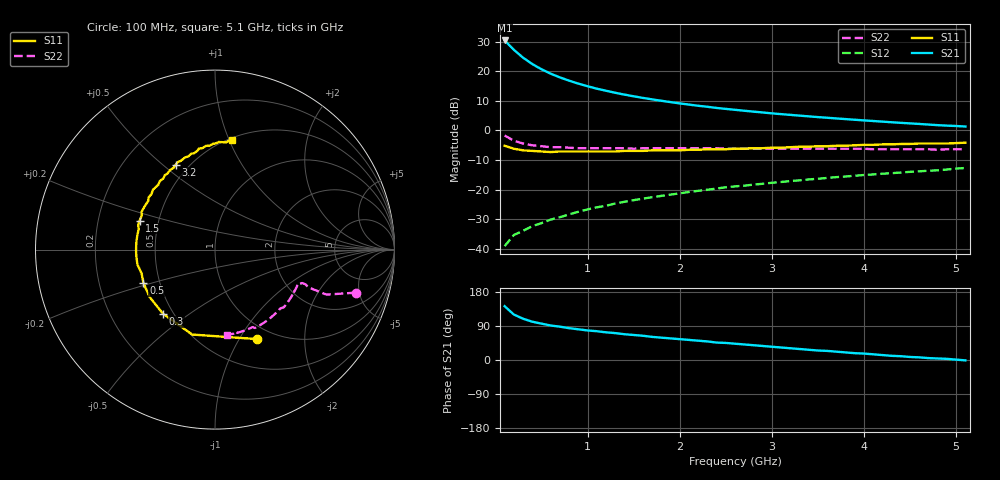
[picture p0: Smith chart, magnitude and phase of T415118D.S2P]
!AT-41511
!S-PARAMETERS at Vce=8V  Ic=25mA.  LAST UPDATED 01-25-95
# ghz s ma r 50
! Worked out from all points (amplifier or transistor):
!   51 points, 100 MHz to 5.1 GHz, reference 50 ohm
!   highest |S21| = 30.4 dB at 100 MHz (marker M1)
!   |S21| within 3 dB of that: start of sweep to 195.3 MHz
!   unconditionally stable (mu >= 1): 646.1 MHz to 3.16 GHz
!   at 900 MHz: K = 1.08, MAG = 20.0 dB, |S12| = -27.5 dB
!   at 2.6 GHz: K = 1.05, MAG = 11.6 dB, |S12| = -18.9 dB
!   at 5.1 GHz: K = 0.81, MSG = 7.0 dB, |S12| = -12.7 dB
!   lowest NFmin = 1.60 dB at 100 MHz
!   S11 on the Smith chart (normalised r, x): 100 MHz: 0.83, -1.19; 300 MHz: 0.44, -0.40; 500 MHz: 0.40, -0.19; 1.5 GHz: 0.39, +0.16; 3.2 GHz: 0.43, +0.55; 5.1 GHz: 0.52, +1.03
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0.1  0.55 -65.0  33.26 142.0  0.011 66.0  0.82 -17.0
0.2  0.49 -105.0  23.16 120.0  0.017 58.0  0.67 -22.0
0.3  0.46 -129.0  17.02 109.0  0.02 57.0  0.6 -22.0
0.4  0.45 -144.0  13.27 101.0  0.024 59.0  0.56 -22.0
0.5  0.44 -155.0  10.83 96.0  0.027 61.0  0.54 -21.0
0.6  0.43 -162.0  9.118 91.0  0.031 62.0  0.52 -21.0
0.7  0.44 -169.0  7.888 88.0  0.034 64.0  0.52 -21.0
0.8  0.44 -175.0  6.943 84.0  0.038 65.0  0.51 -22.0
0.9  0.44 -179.0  6.19 81.0  0.042 66.0  0.5 -22.0
1  0.44 176.0  5.588 78.0  0.046 67.0  0.5 -23.0
1.1  0.44 173.0  5.085 76.0  0.05 67.0  0.5 -24.0
1.2  0.44 169.0  4.689 73.0  0.053 67.0  0.5 -25.0
1.4  0.45 162.0  4.035 68.0  0.062 67.0  0.5 -28.0
1.5  0.45 159.0  3.779 66.0  0.066 67.0  0.49 -29.0
1.8  0.46 150.0  3.173 59.0  0.078 67.0  0.5 -32.0
2  0.46 144.0  2.865 55.0  0.086 66.0  0.5 -35.0
2.4  0.48 133.0  2.401 46.0  0.104 65.0  0.5 -40.0
2.6  0.49 129.0  2.23 43.0  0.113 64.0  0.49 -43.0
3.2  0.52 115.0  1.832 31.0  0.139 60.0  0.49 -51.0
3.5  0.54 108.0  1.68 25.0  0.152 58.0  0.49 -55.0
4.3  0.58 93.0  1.374 11.0  0.189 53.0  0.48 -68.0
5.1  0.62 81.0  1.164 -1.0  0.231 47.0  0.48 -82.0
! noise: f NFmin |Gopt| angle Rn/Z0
0.1  1.6  0.08  10  0.2
0.9  1.9  0.1  100  0.19
1.8  2.3  0.22  -170  0.18
2.4  2.7  0.32  -147  0.18
